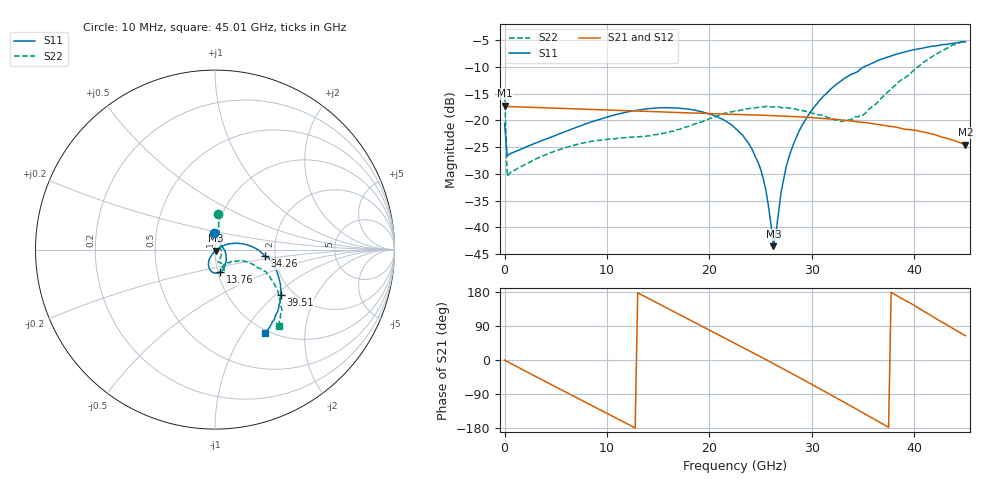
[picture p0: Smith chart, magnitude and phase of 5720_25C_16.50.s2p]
! Device:  ADRF5720
! Description: 0.5dB LSB GaAs MMIC 6-bit Digital Attenuator
! Frequency:  0.000009 -  40 GHz
! Ports:
!	RF1	= Port 1
!	RF2	= Port 2
! Vdd:  3.3 Volt
! Vss:  -3.3 Volt
! Control:  0/3.3 Volt
! State:  16.50 dB attenuation
! Data:  The device was measured using G-S-G Probes on a matrix board.
!  Data was collected using an calibrated 4 port network analyzer.
!  The reference plane for this measurement is at the launchers.
! Note:  Analog Devices supplies this data as a sample of measured data
!  for this product.  Your particular data for this product may vary.
!  Data was taken at 25 degrees C.
!  Analog Devices reserves the right to change this data at anytime.
# GHZ S DB R 45.0
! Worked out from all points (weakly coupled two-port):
!   181 points, 10 MHz to 45.01 GHz, reference 45 ohm
!   highest |S21| = -17.22 dB at 10 MHz (marker M1); lowest = -24.5 dB at 45.01 GHz (marker M2)
!   lowest |S11| = -43.5 dB at 26.26 GHz (marker M3), VSWR 1.01, Z = 45.3 - j0.525 ohm
!   |S11| at or under -10 dB: start of sweep to 35.1 GHz
!   |S22| runs from -30.5 to -5.1 dB; largest |S21 - S12| = 0.00031
!   S11 on the Smith chart (normalised r, x): 10 MHz: 0.97, +0.18; 13.76 GHz: 1.02, -0.26; 34.26 GHz: 1.76, -0.14; 39.51 GHz: 1.72, -1.09; 45.01 GHz: 0.95, -1.26
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0.01  -20.59 94.7  -17.22 -0.2  -17.21 -0.1  -13.92 85.3
0.26  -26.65 10.3  -17.40 -3.9  -17.41 -3.9  -30.46 14.9
3.51  -23.88 -20.7  -17.62 -50.1  -17.62 -50.1  -26.82 -37.8
7.76  -20.77 -47.9  -17.90 -109.5  -17.90 -109.5  -24.18 -67.9
13.76  -17.88 -77.3  -18.30 166.8  -18.31 166.8  -22.96 -74.0
15.26  -17.63 -83.9  -18.39 145.6  -18.40 145.7  -22.52 -70.8
20.26  -18.91 -105.2  -18.74 75.5  -18.74 75.6  -19.53 -62.8
22.76  -21.83 -116.5  -18.90 40.4  -18.90 40.4  -18.22 -65.4
24.01  -24.85 -121.3  -18.98 22.7  -18.99 22.7  -17.73 -67.9
25.01  -29.12 -121.3  -19.02 8.5  -19.02 8.5  -17.47 -69.8
25.51  -32.89 -115.9  -19.05 1.3  -19.06 1.3  -17.39 -71.3
26.26  -43.50 -60.1  -19.11 -9.5  -19.11 -9.5  -17.47 -71.4
27.01  -33.42 18.4  -19.16 -20.4  -19.16 -20.3  -17.60 -73.6
27.76  -26.96 26.3  -19.24 -31.3  -19.24 -31.2  -17.69 -74.2
28.76  -22.02 22.9  -19.33 -45.8  -19.33 -45.7  -18.08 -75.5
30.26  -17.45 15.2  -19.51 -68.0  -19.51 -68.0  -18.73 -73.4
32.76  -12.78 1.2  -19.88 -105.4  -19.89 -105.3  -20.20 -59.9
34.26  -11.09 -7.5  -20.20 -128.0  -20.20 -127.9  -19.29 -42.7
37.76  -7.94 -25.9  -21.12 178.7  -21.13 178.8  -14.18 -20.6
39.51  -7.01 -34.9  -21.73 152.0  -21.73 152.1  -11.56 -23.0
42.01  -6.10 -46.5  -22.65 111.3  -22.64 111.4  -7.74 -32.5
45.01  -5.31 -59.3  -24.51 64.3  -24.51 64.3  -5.06 -50.1
